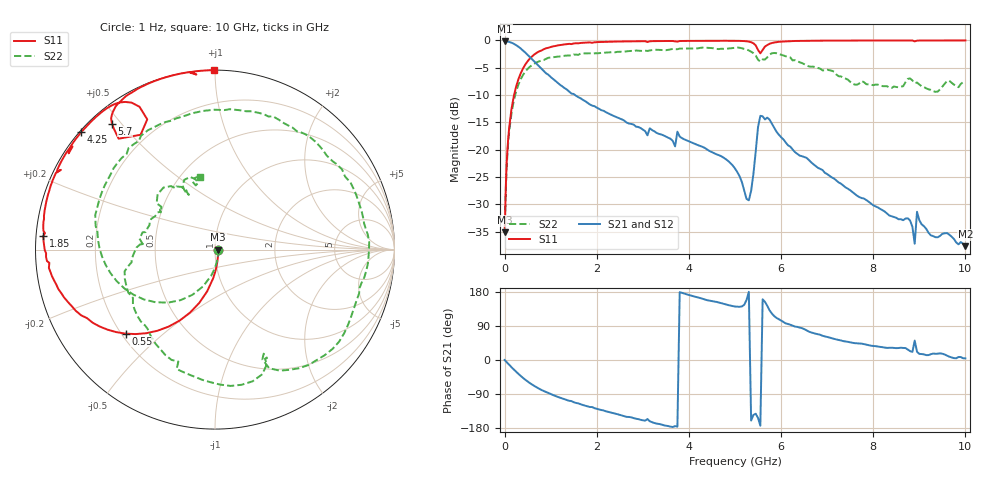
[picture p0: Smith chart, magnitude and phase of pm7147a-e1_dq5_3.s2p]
# GHz S DB R 50
! S-Parameters data
! Freq  dbS11  angS11  dbS21  angS21  dbS12  angS12  dbS22  angS22
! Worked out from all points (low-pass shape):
!   279 points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, 1 Hz to 10 GHz, reference 50 ohm
!   highest |S21| = -0.15 dB at 19.95 kHz (marker M1); lowest = -37.7 dB at 10 GHz (marker M2)
!   |S21| within 3 dB of the highest: start of sweep to 561.6 MHz
!   lowest |S11| = -35.1 dB at 15.85 kHz (marker M3), VSWR 1.04, Z = 51.8 - j0.00241 ohm
!   |S11| at or under -10 dB: start of sweep to 205.3 MHz
!   |S22| runs from -35.1 to -1.3 dB; largest |S21 - S12| = 0
!   S11 on the Smith chart (normalised r, x): 1 Hz: 1.04, -0.00; 550 MHz: 0.22, -0.38; 1.85 GHz: 0.02, +0.04; 4.25 GHz: 0.00, +0.38; 5.7 GHz: 0.06, +0.47; 10 GHz: 0.00, +0.99
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1e-09  -35.08 -0.0  -0.15 -0.0  -0.15 -0.0  -35.08 -0.0
1.58489e-05  -35.08 -0.1  -0.15 -0.0  -0.15 -0.0  -35.08 -0.1
1.99526e-05  -35.08 -0.1  -0.15 -0.0  -0.15 -0.0  -35.08 -0.1
0.05011872  -21.67 -82.5  -0.19 -6.4  -0.19 -6.4  -22.38 -84.1
0.15  -12.52 -100.6  -0.42 -19.0  -0.42 -19.0  -13.30 -108.1
0.55  -3.30 -136.8  -3.06 -61.1  -3.06 -61.1  -4.81 -162.2
0.95  -1.34 -158.3  -6.28 -86.9  -6.28 -86.9  -3.17 163.9
1.7  -0.43 178.9  -10.89 -118.9  -10.89 -118.9  -2.35 119.4
1.85  -0.36 175.5  -11.72 -124.1  -11.72 -124.1  -2.35 111.2
3.35  -0.11 150.5  -17.11 -168.8  -17.11 -168.8  -1.73 44.7
4.25  -0.07 138.6  -19.33 163.3  -19.33 163.3  -1.36 5.6
5.05  -0.07 127.9  -24.10 140.7  -24.10 140.7  -1.30 -36.6
5.3  -0.22 122.8  -29.26 180.0  -29.26 180.0  -1.84 -54.8
5.55  -2.36 122.9  -13.80 -173.5  -13.80 -173.5  -3.87 -64.9
5.7  -0.85 129.3  -14.13 143.0  -14.13 143.0  -3.08 -65.7
5.95  -0.25 124.7  -17.24 107.7  -17.24 107.7  -2.47 -87.9
6.7  -0.05 115.8  -22.66 71.1  -22.66 71.1  -4.80 -135.8
8.35  -0.01 101.5  -32.05 32.2  -32.05 32.2  -8.64 145.1
8.8  -0.01 98.0  -32.97 23.4  -32.97 23.4  -6.95 129.7
8.9  -0.17 96.1  -37.21 51.3  -37.21 51.3  -7.83 122.6
8.95  -0.04 98.0  -31.36 21.8  -31.36 21.8  -7.70 121.4
10  -0.00 90.4  -37.66 4.4  -37.66 4.4  -7.63 101.8
